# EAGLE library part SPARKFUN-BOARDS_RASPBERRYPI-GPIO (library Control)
RASPBERRY PI I/O HEADER As defined for the Revistion 2 Pi.
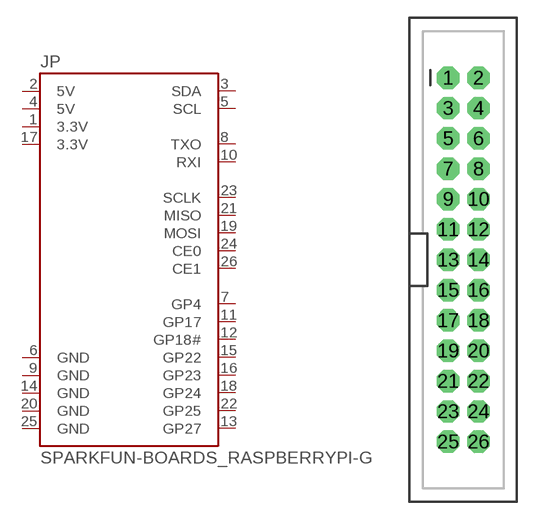
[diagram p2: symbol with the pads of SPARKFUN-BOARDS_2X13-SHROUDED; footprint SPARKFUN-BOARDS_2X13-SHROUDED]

Designator prefix JP

## SPARKFUN-BOARDS_RASPBERRYPI-GPIOPTH (DIST: sparkfun; DIST_ID: PRT-11490)  [SPARKFUN-BOARDS_2X13-SHROUDED]
1  3.3V  pwr
2  5V  pwr
3  SDA
4  5V  pwr
5  SCL
6  GND  pwr
7  GP4
8  TXO  out
9  GND  pwr
10  RXI  in
11  GP17
12  GP18#
13  GP27
14  GND  pwr
15  GP22
16  GP23
17  3.3V  pwr
18  GP24
19  MOSI  out
20  GND  pwr
21  MISO  in
22  GP25
23  SCLK  out
24  CE0  out
25  GND  pwr
26  CE1  out

## Footprint SPARKFUN-BOARDS_2X13-SHROUDED (pad centres in mm)
drill 1.016 pad 1.88 octagon: 1 -1.27,15.24; 2 1.27,15.24; 3 -1.27,12.7; 4 1.27,12.7; 5 -1.27,10.16; 6 1.27,10.16; 7 -1.27,7.62; 8 1.27,7.62; 9 -1.27,5.08; 10 1.27,5.08; 11 -1.27,2.54; 12 1.27,2.54; 13 -1.27,0; 14 1.27,0; 15 -1.27,-2.54; 16 1.27,-2.54; 17 -1.27,-5.08; 18 1.27,-5.08; 19 -1.27,-7.62; 20 1.27,-7.62; 21 -1.27,-10.16; 22 1.27,-10.16; 23 -1.27,-12.7; 24 1.27,-12.7; 25 -1.27,-15.24; 26 1.27,-15.24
